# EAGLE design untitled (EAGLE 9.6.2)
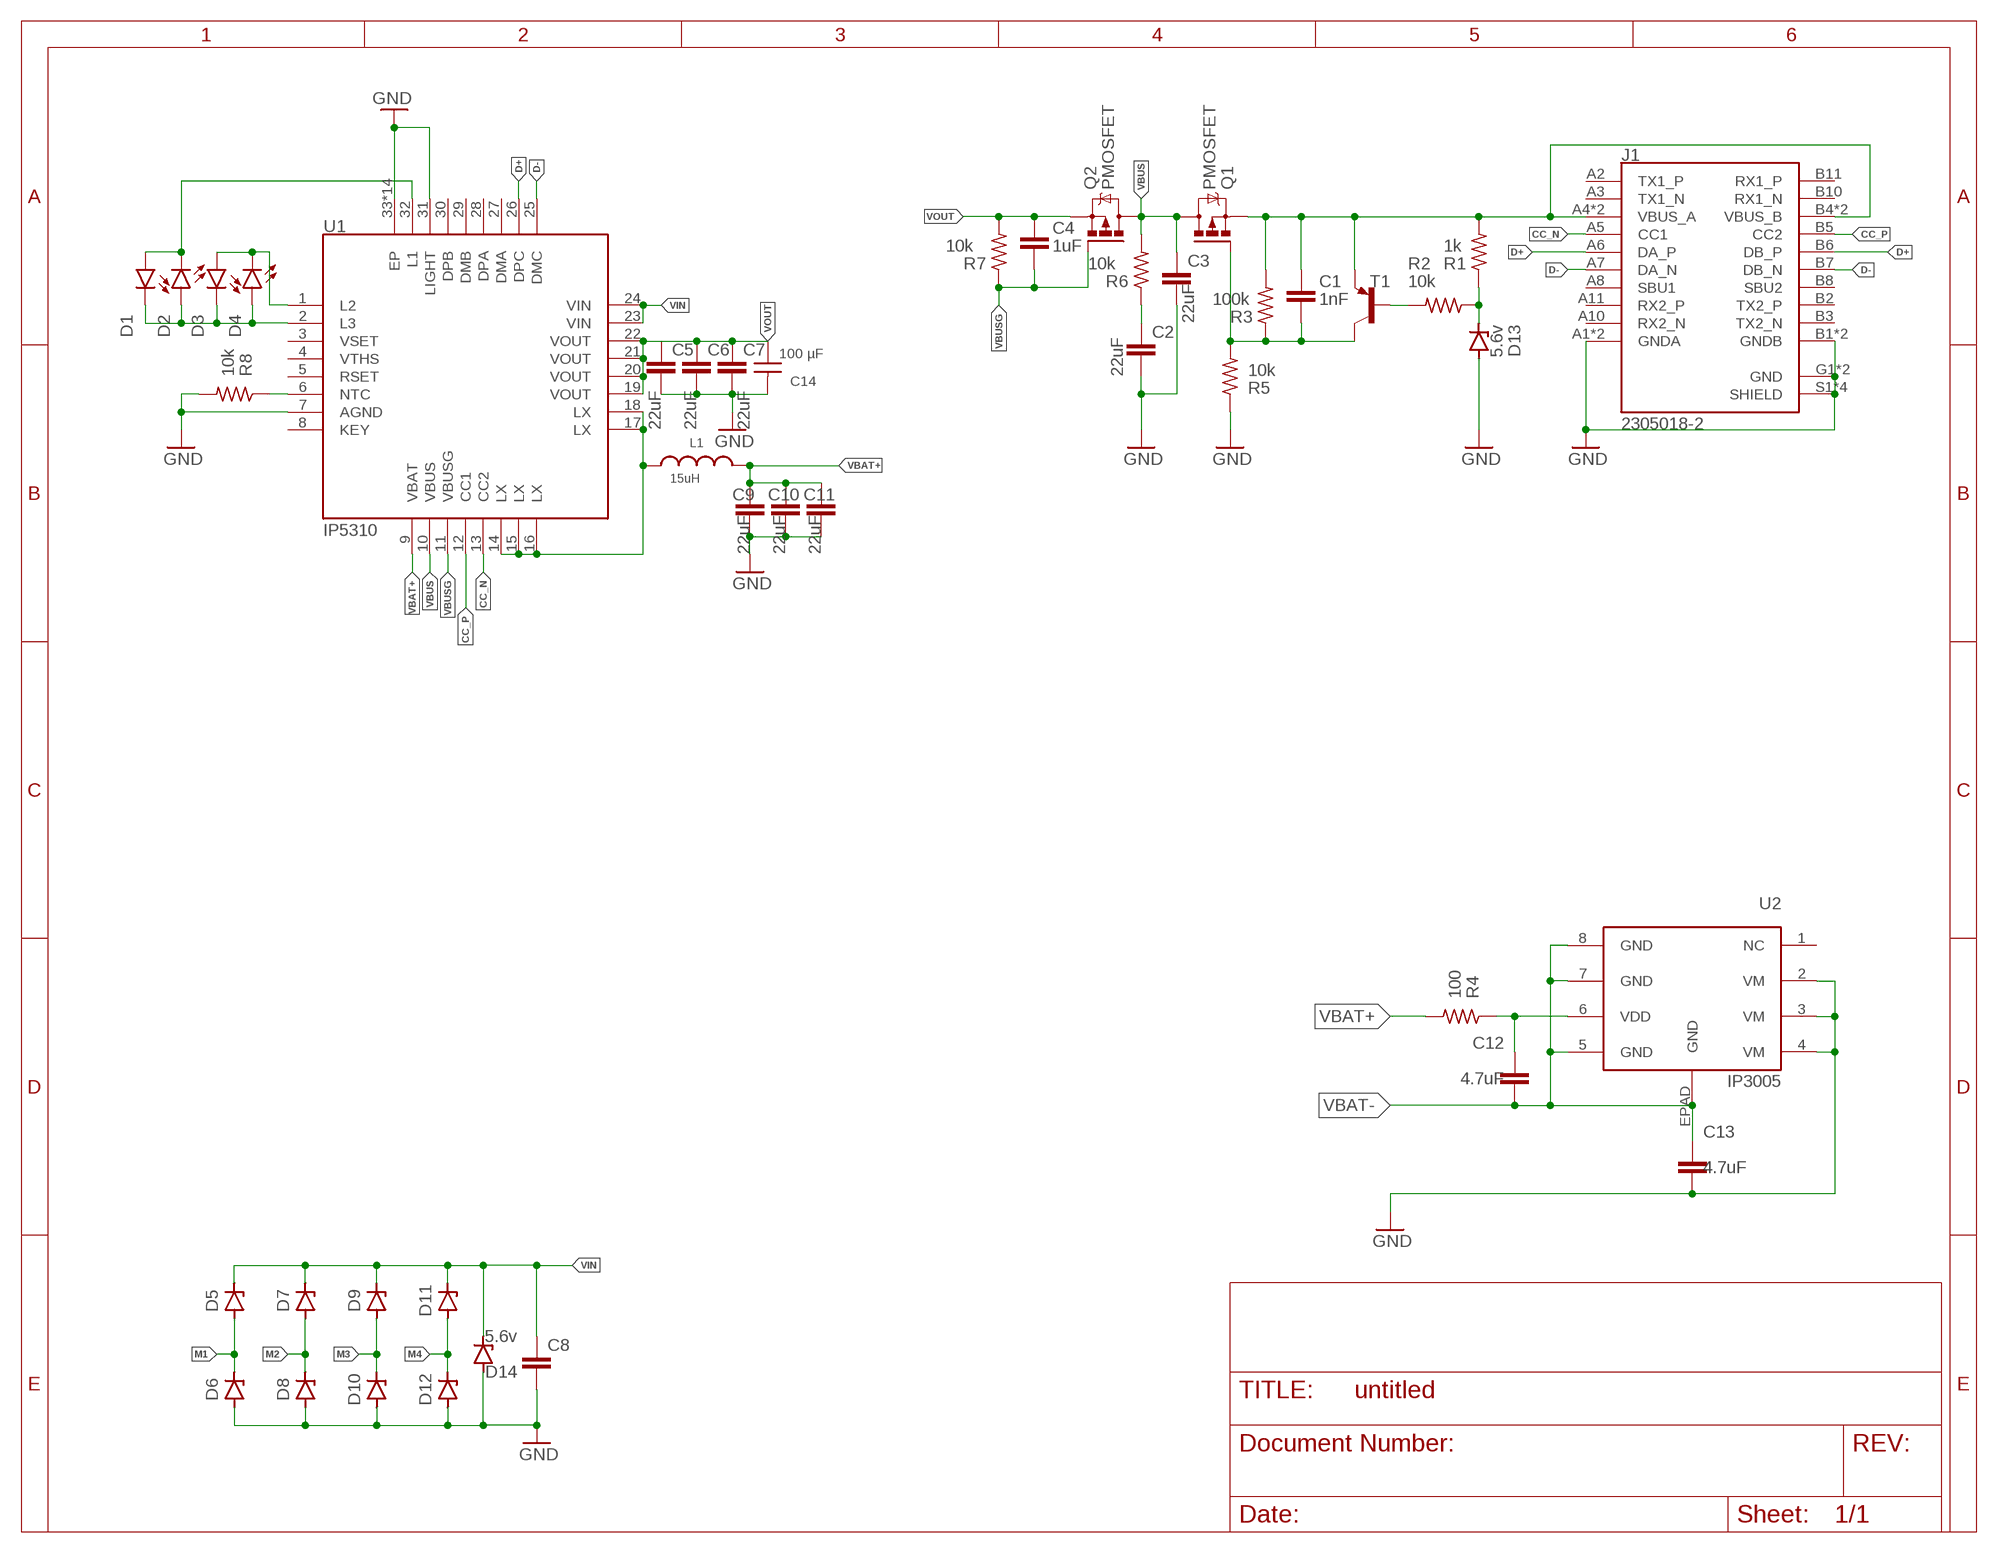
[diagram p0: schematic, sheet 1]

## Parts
C1  1nF  CC0603JRNPO9BN220  [CAP_0603]
C2  22uF  C-EUC0805  [C0805]
C3  22uF  C-EUC0805  [C0805]
C4  1uF  CC0603JRNPO9BN220  [CAP_0603]
C5  22uF  C-EUC0805  [C0805]
C6  22uF  C-EUC0805  [C0805]
C7  22uF  C-EUC0805  [C0805]
C8  C-EUC0805  [C0805]
C9  22uF  C-EUC0805  [C0805]
C10  22uF  C-EUC0805  [C0805]
C11  22uF  C-EUC0805  [C0805]
C12  4.7uF  C0603C120J5GACTU  [CAP_0603]
C13  4.7uF  C0603C120J5GACTU  [CAP_0603]
C14  100 µF  WCAP-ASNP_6.3X5.5_865250143004  [WCAP-ASNP_6.3X5.5(DXL)]
D1  LEDCHIPLED_0603  [CHIPLED_0603]
D2  LEDCHIPLED_0603  [CHIPLED_0603]
D3  LEDCHIPLED_0603  [CHIPLED_0603]
D4  LEDCHIPLED_0603  [CHIPLED_0603]
D5  ZENER_MMSZ5240BTDO-219-AB(SOD123F)  [SODFL3718X115]
D6  ZENER_MMSZ5240BTDO-219-AB(SOD123F)  [SODFL3718X115]
D7  ZENER_MMSZ5240BTDO-219-AB(SOD123F)  [SODFL3718X115]
D8  ZENER_MMSZ5240BTDO-219-AB(SOD123F)  [SODFL3718X115]
D9  ZENER_MMSZ5240BTDO-219-AB(SOD123F)  [SODFL3718X115]
D10  ZENER_MMSZ5240BTDO-219-AB(SOD123F)  [SODFL3718X115]
D11  ZENER_MMSZ5240BTDO-219-AB(SOD123F)  [SODFL3718X115]
D12  ZENER_MMSZ5240BTDO-219-AB(SOD123F)  [SODFL3718X115]
D13  5.6v  ZENER_MMSZ5240BTDO-219-AB(SOD123F)  [SODFL3718X115]
D14  5.6v  ZENER_MMSZ5240BTDO-219-AB(SOD123F)  [SODFL3718X115]
J1  2305018-2  [TE_2305018-2]
L1  15uH  WE-LHMI_7050_74437349150  [WE-LHMI_7050]
Q1  PMOSFET  PMOSFET_SOT23  [SOT23]
Q2  PMOSFET  PMOSFET_SOT23  [SOT23]
R1  1k  RC0603JR-070RL  [RES_0603]
R2  10k  RC0603JR-070RL  [RES_0603]
R3  100k  RC0603JR-070RL  [RES_0603]
R4  100  RC0603JR-070RL  [RES_0603]
R5  10k  RC0603JR-070RL  [RES_0603]
R6  10k  RC0603JR-070RL  [RES_0603]
R7  10k  RC0603JR-070RL  [RES_0603]
R8  10k  RC0603JR-070RL  [RES_0603]
T1  BC808-16-PNP-SOT23-BEC  [SOT23-BEC]
U1  IP5310  [VQFN_32]
U2  IP3005  [HSOP8]

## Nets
CC_N [cc lines]: J1.A5(CC1) U1.13(CC2)
CC_P [cc lines]: J1.B5(CC2) U1.12(CC1)
D+: J1.A6(DA_P) J1.B6(DB_P) U1.26(DPC)
D-: J1.A7(DA_N) J1.B7(DB_N) U1.25(DMC)
GND: C2.2 C3.2 C5.2 C6.2 C7.2 C8.2 C9.2 C10.2 C11.2 C13.2 C14.2 D6.2(A) D8.2(A) D10.2(A) D12.2(A) D13.2(A) D14.2(A) J1.A1(GNDA) J1.A12(GNDA) J1.B1(GNDB) J1.B12(GNDB) J1.G1(GND) J1.G2(GND) J1.S1(SHIELD) J1.S2(SHIELD) J1.S3(SHIELD) J1.S4(SHIELD) R5.1 R8.2 U1.7(AGND) U1.31(LIGHT) U1.33(EP) U1.P$1(EP) U1.P$2(EP) U1.P$3(EP) U1.P$4(EP) U1.P$5(EP) U1.P$6(EP) U1.P$7(EP) U1.P$8(EP) U1.P$9(EP) U1.P$10(EP) U1.P$11(EP) U1.P$12(EP) U1.P$13(EP) U2.2(VM) U2.3(VM) U2.4(VM)
M1: D5.2(A) D6.1(C)
M2: D7.2(A) D8.1(C)
M3: D9.2(A) D10.1(C)
M4: D11.2(A) D12.1(C)
N$1: C1.1 J1.A4(VBUS_A) J1.A9(VBUS_A) J1.B4(VBUS_B) J1.B9(VBUS_B) Q1.2(S) R1.2 R3.2 T1.E
N$2: R8.1 U1.6(NTC)
N$3: L1.1 U1.14(LX) U1.15(LX) U1.16(LX) U1.17(LX) U1.18(LX)
N$6: C2.1 R6.1
N$8: C1.2 Q1.1(G) R3.1 R5.2 T1.C
N$9: R2.2 T1.B
N$10: D1.A D2.C U1.32(L1)
N$11: D3.A D4.C U1.1(L2)
N$12: C12.1 R4.1 U2.6(VDD)
N$13: D1.C D2.A D3.C D4.A U1.2(L3)
N$14: D13.1(C) R1.1 R2.1
VBAT+: C9.1 C10.1 C11.1 L1.2 R4.2 U1.9(VBAT)
VBAT-: C12.2 C13.1 U2.5(GND) U2.7(GND) U2.8(GND) U2.EPAD(GND)
VBUS: C3.1 Q1.3(D) Q2.3(D) R6.2 U1.10(VBUS)
VBUSG: C4.2 Q2.1(G) R7.1 U1.11(VBUSG)
VIN: C8.1 D5.1(C) D7.1(C) D9.1(C) D11.1(C) D14.1(C) U1.23(VIN) U1.24(VIN)
VOUT: C4.1 C5.1 C6.1 C7.1 C14.1 Q2.2(S) R7.2 U1.19(VOUT) U1.20(VOUT) U1.21(VOUT) U1.22(VOUT)
Unconnected: J1.A2(TX1_P) J1.A3(TX1_N) J1.A8(SBU1) J1.A10(RX2_N) J1.A11(RX2_P) J1.B2(TX2_P) J1.B3(TX2_N) J1.B8(SBU2) J1.B10(RX1_N) J1.B11(RX1_P) U1.3(VSET) U1.4(VTHS) U1.5(RSET) U1.8(KEY) U1.27(DMA) U1.28(DPA) U1.29(DMB) U1.30(DPB) U2.1(NC)

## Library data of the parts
C1 C4 = Resistor_Capacitor:CC0603JRNPO9BN220: CAP CER 22PF 50V C0G/NPO 0603; CREATED_BY: PCBLayout.com; DIGIKEY_PART_NUMBER: 311-1062-2-ND; MANUFACTURER: Yageo; MPN: CC0603JRNPO9BN220; PACKAGE: SMD 0603
C2 C3 C5-C11 = resistor:C-EU: CAPACITOR, European symbol
C12 C13 = Resistor_Capacitor:C0603C120J5GACTU: CAP CER 12PF 50V C0G/NP0 0603; CREATED_BY: PCBLayout.com; DIGIKEY_PART_NUMBER: 399-1050-2-ND; MANUFACTURER: KEMET; MPN: C0603C120J5GACTU; PACKAGE: SMD 0603
C14 = Wurth_Capacitors_WCAP-ASNP:WCAP-ASNP_6.3X5.5: WCAP-ASNP Aluminium Electrolytic Capacitors; DATASHEET-URL: https://www.we-online.com/catalog/datasheet/865250143004.pdf; DF: 24%; DIAMETER: 6.3mm; I-LEAK: 14.805uA; I-RIPPLE: 45mA; L: 5.5mm; OPERATING-TEMPERATURE: -40 °C up to +85 °C; PART-NUMBER: 865250143004; TECHNICAL-REFERENCE: ASBD055470M6R3DVCTBB000; VALUE: 47 µF; VR: 6.3V(DC); Z: 0.990213Ohm
D1-D4 = led:LED: LED
D5-D14 = Diode:ZENER_: Zener Diode - Popular parts; CATEGORY: Diode; DESCRIPTION: DIODE ZENER 10V 500MW SOD123; MANUFACTURER: ON Semiconductor; MPN: MMSZ5240BT1G; SUB-CATEGORY: Zener; THERMALLOSS: 0.5W; VALUE: MMSZ5240BT1G
J1 = type-c:2305018-2: TYPE C Right Angle Sealable SMT IPX8 3.1 GEN 2 Wire to Board USB; COMMENT: 2305018-2; DESCRIPTION: USB TYPE C, REC IPX8 ON BOARD DUAL SMT; DIGI-KEY_PART_NUMBER: A132569CT-ND; MF: TE Connectivity; MP: 2305018-2; PACKAGE: None; PURCHASE-URL: https://pricing.snapeda.com/search/part/2305018-2/?ref=eda
L1 = Wurth_Power Magnetics_WE-LHMI:WE-LHMI_7050: WE-LHMI SMD Power Inductor; DATASHEET-URL: https://www.we-online.com/catalog/datasheet/74437349150.pdf; FRES: 10MHz; IR: 2.75A; ISAT: 5.5A; MOUNT: SMT; PART-NUMBER: 74437349150; RDC-MAX: 92mOhm; RDC-TYPE: 81mOhm
Q1 Q2 = Transistor:PMOSFET: P-Channel MOSFET - Generic; CATEGORY: Transistor; SUB-CATEGORY: MOSFET; TYPE: P-Channel
R1-R8 = Resistor_Capacitor:RC0603JR-070RL: RES SMD 0 OHM JUMPER 1/10W 0603; CREATED_BY: PCBLayout.com; DIGIKEY_PART_NUMBER: 311-0.0GRTR-ND; MANUFACTURER: Yageo; MPN: RC0603JR-070RL; PACKAGE: SMD 0603
T1 = transistor-neu-to92:*-PNP-: PNP Transistror
U1 = INJOINIC:IP5310
U2 = INJOINIC:IP3005

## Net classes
1 cc lines: width 0.203 mm, clearance 0.152 mm

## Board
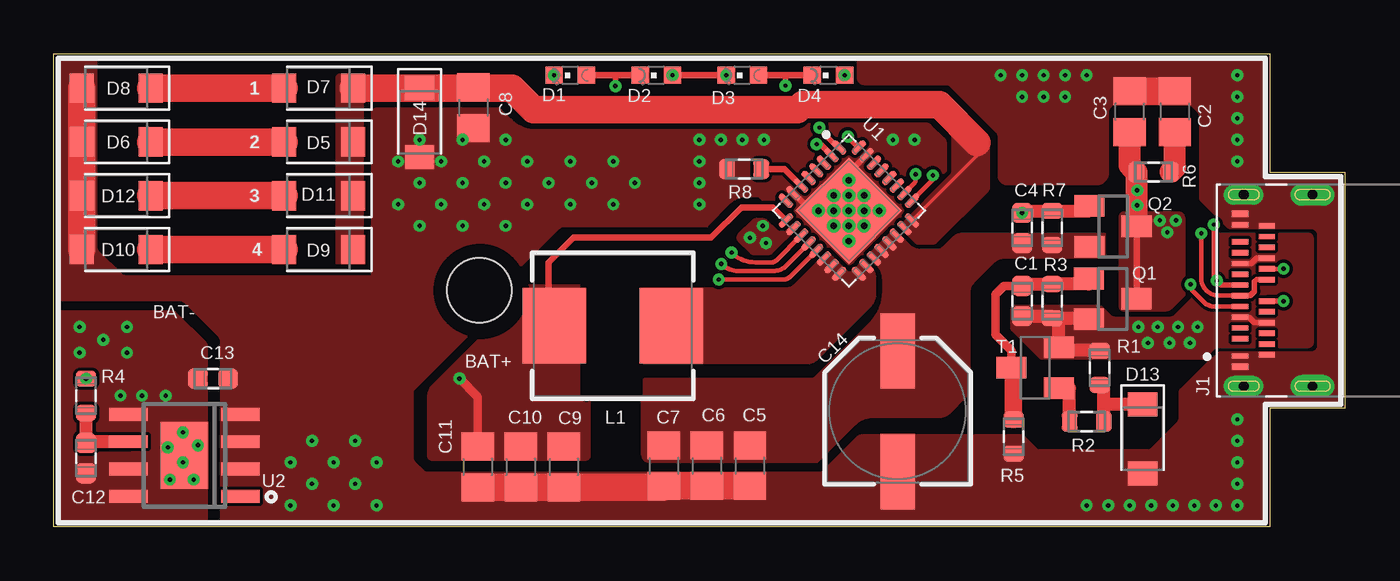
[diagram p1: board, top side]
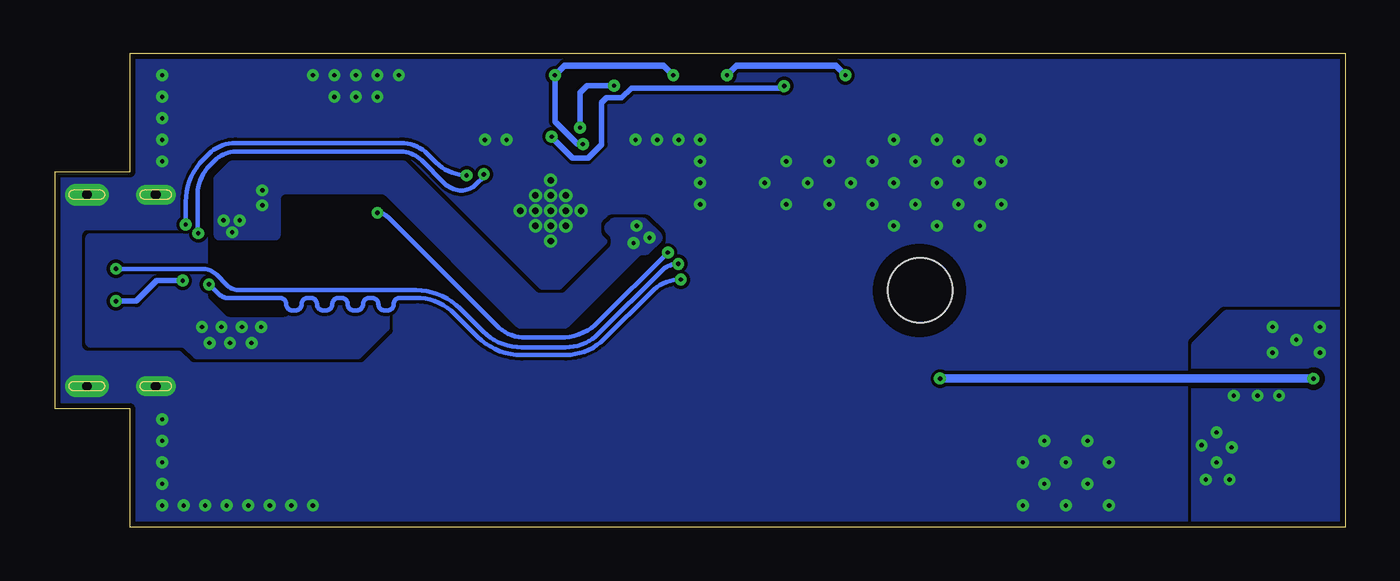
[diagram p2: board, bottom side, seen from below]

Size 60 x 22 mm. Coordinates in mm from the lower left corner, seen from the top.
Outline: 0,0 0,22 56.5,22 56.5,16.5 60,16.5 60,5.5 56.5,5.5 56.5,0 0,0
Copper layers (1*16): Top 0.035mm / dielectric 1.5mm / Bottom 0.035mm
Design rules "default *": minimum track width 6mil, minimum drill 0.1mm, track to track 6mil, track to pad 6mil, pad to pad 6mil, via to via 6mil, smd to smd 0mil, copper to edge 10mil, drill to drill 3mil, minimum pad ring 3mil, minimum via ring 3mil, stop-mask expansion 0mil, vias tented up to drill 1mm, thermal gap 10mil
Holes 3 mm at 19.78,11
tRestrict: area 53.5,11.4 to 53.6,13.3; area 52.8,11.7 to 53.1,13.6; area 18.3,9.5 to 21.3,12.5
bRestrict: area 18.3,9.5 to 21.3,12.5

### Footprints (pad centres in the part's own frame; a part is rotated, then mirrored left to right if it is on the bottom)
CAP_0603 = smd 0.92 x 0.93: 1 -0.705,0; 2 0.705,0
C0805 = smd 1.3 x 1.5: 1 -0.95,0; 2 0.95,0
WCAP-ASNP_6.3X5.5(DXL) = smd 3.5 x 1.6: 1 2.8,0; 2 -2.8,0
CHIPLED_0603 = smd 0.8 x 0.8: A 0,-0.75; C 0,0.75
SODFL3718X115 = smd 1.115 x 1.361: 1 -1.6,0; 2 1.6,0
TE_2305018-2 = smd 0.25 x 0.75: A1 -3.05,3.375; A2 -2.25,3.375; A3 -1.75,3.375; A4 -1.25,3.375; A5 -0.75,3.375; A6 -0.25,3.375; A7 0.25,3.375; A8 0.75,3.375; A9 1.25,3.375; A10 1.75,3.375; A11 2.25,3.375; A12 3.05,3.375; B1 3,2.125; B2 2.5,2.125; B3 2,2.125; B4 1.5,2.125; B5 1,2.125; B6 0.5,2.125; B7 -0.5,2.125; B8 -1,2.125; B9 -1.5,2.125; B10 -2,2.125; B11 -2.5,2.125; B12 -3,2.125 | smd 0.3 x 0.75: G1 -3.55,3.375; G2 3.55,3.375 | drill 0.45 pad 1.025 long: S1 -4.45,0; S2 4.45,0 | drill 0.45 pad 0.925 long: S3 -4.45,3.2; S4 4.45,3.2
WE-LHMI_7050 = smd 2.95 x 3.5: 1 -2.725,0; 2 2.725,0
SOT23 = smd 1 x 1.4: 1 -0.95,-1.1; 2 0.95,-1.1; 3 0,1.1
RES_0603 = smd 0.74 x 0.93: 1 -0.795,0; 2 0.795,0
SOT23-BEC = smd 1 x 1.4: B -0.95,-1.1; C 0,1.1; E 0.95,-1.1
VQFN_32 = smd 0.8 x 0.3: 1 -2.4,1.75; 2 -2.4,1.25; 3 -2.4,0.75; 4 -2.4,0.25; 5 -2.4,-0.25; 6 -2.4,-0.75; 7 -2.4,-1.25; 8 -2.4,-1.75; 17 2.4,-1.75; 18 2.4,-1.25; 19 2.4,-0.75; 20 2.4,-0.25; 21 2.4,0.25; 22 2.4,0.75; 23 2.4,1.25; 24 2.4,1.75 | smd 0.3 x 0.8: 9 -1.75,-2.4; 10 -1.25,-2.4; 11 -0.75,-2.4; 12 -0.25,-2.4; 13 0.25,-2.4; 14 0.75,-2.4; 15 1.25,-2.4; 16 1.75,-2.4; 25 1.75,2.4; 26 1.25,2.4; 27 0.75,2.4; 28 0.25,2.4; 29 -0.25,2.4; 30 -0.75,2.4; 31 -1.25,2.4; 32 -1.75,2.4 | smd 3.5 x 3.5: 33 0,0 | drill 0.3 pad 0.61: P$1 -1,1; P$2 0,1; P$3 1,1; P$4 -0.5,0.5; P$5 0.5,0.5; P$6 -1,0; P$7 0,0; P$8 1,0; P$9 -0.5,-0.5; P$10 0.5,-0.5; P$11 -1,-1; P$12 0,-1; P$13 1,-1
HSOP8 = smd 1.8 x 0.6: 1 -2.6,1.905; 2 -2.6,0.635; 3 -2.6,-0.635; 4 -2.6,-1.905; 5 2.6,-1.905; 6 2.6,-0.635; 7 2.6,0.635; 8 2.6,1.905 | smd 2.21 x 3.1: EPAD 0,0

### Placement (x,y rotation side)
C1  45,10.5 90 top
C2  52.1,19.3 90 top
C3  50,19.3 90 top
C4  45,13.9 90 top
C5  32.35,2.85 270 top
C6  30.35,2.85 270 top
C7  28.35,2.85 270 top
C8  19.5,19.5 270 top
C9  23.7,2.8 270 top
C10  21.7,2.8 270 top
C11  19.7,2.8 270 top
C12  1.5,3.2 270 top
C13  7.4,6.9 0 top
C14  39.21,5.38 90 top
D1  24,21 90 top
D2  28,21 90 top
D3  32,21 90 top
D4  36,21 90 top
D5  12.3,17.9 180 top
D6  2.9,17.9 180 top
D7  12.3,20.4 180 top
D8  2.9,20.4 180 top
D9  12.3,12.9 180 top
D10  2.9,12.9 180 top
D11  12.3,15.4 180 top
D12  2.9,15.4 180 top
D13  50.6,4.1 270 top
D14  17,18.8 270 top
J1  58.5,11 90 top
L1  25.98,9.36 180 top
Q1  49.2,10.6 270 top
Q2  49.22,13.97 270 top
R1  48.6,7.4 90 top
R2  48,4.9 180 top
R3  46.4,10.5 270 top
R4  1.5,6.1 90 top
R5  44.6,4.2 90 top
R6  51.1,16.5 180 top
R7  46.4,13.9 270 top
R8  32.08,16.64 180 top
T1  45.6,7.4 90 top
U1  36.95,14.71 315 top
U2  6.07,3.33 180 top

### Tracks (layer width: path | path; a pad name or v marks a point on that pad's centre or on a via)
CC_N  (via drill 0.2 pad 0.55)
  Top 0.203: U1.13 34.24,11.64 arc-45 33.9,11.5 v30.9,11.5 | J1.A5 53.93,10.25 arc-45 53.45,10.45 52.97,10.93 arc-45 v52.83,11.28
  Bottom 0.203: v30.9,11.5 arc-45 32.27,10.93 34.47,8.73 arc45 36.25,7.99 38.3,7.99 arc45 40.34,8.84 41.41,9.91 arc-45 43.2,10.65 43.95,10.65 arc-90 44.24,10.36 arc90 44.53,10.07 44.66,10.07 arc90 44.95,10.36 arc-90 45.25,10.65 45.38,10.65 arc-90 45.67,10.36 arc90 45.96,10.07 46.09,10.07 arc90 46.38,10.36 arc-90 46.67,10.65 46.8,10.65 arc-90 47.09,10.36 arc90 47.39,10.07 47.52,10.07 arc90 47.81,10.36 arc-90 48.1,10.65 48.23,10.65 arc-90 48.52,10.36 arc90 48.81,10.07 48.94,10.07 arc90 49.23,10.36 arc-90 49.53,10.65 51.93,10.65 arc-45 51.94,10.64 arc45 52.37,10.82 v52.83,11.28
CC_P  (via drill 0.2 pad 0.55)
  Top 0.203: v57.15,12 J1.B5 | U1.12 34.03,12.14 arc-45 33.45,11.9 31.81,11.9 arc-45 v31.01,12.23
  Bottom 0.203: v31.01,12.23 arc-45 31.8,11.9 34.72,8.98 arc45 36.25,8.35 38.3,8.35 arc45 40.09,9.09 41.16,10.16 arc-45 43.2,11.01 51.41,11.01 arc45 52,11.25 52.48,11.73 arc-45 53.14,12 v57.15,12
D+  (via drill 0.2 pad 0.55)
  Top 0.203: J1.A6 54.15,10.75 arc-90 53.32,11.58 v53.32,13.65 | v40.05,16.4 40.05,16.16 arc-45 39.97,15.95 U1.26
  Top 0.254: J1.A6 55.6,10.75 55.8,10.95 55.8,11.4 55.9,11.5 J1.B6
  Bottom 0.203: v53.32,13.65 53.35,13.68 53.35,15.47 arc45 52.8,16.8 52.55,17.05 arc45 51.6,17.45 43.9,17.45 arc45 42.95,17.05 41.87,15.97 arc-45 41.09,15.64 arc-45 40.44,15.91 40.05,16.3 v40.05,16.4
D-  (via drill 0.2 pad 0.55)
  Top 0.203: v53.91,14.06 53.9,14.05 53.9,11.81 arc45 v54.05,11.45 | v40.85,16.35 arc-45 40.7,15.98 U1.25
  Top 0.254: J1.A7 54.25,11.25 v54.05,11.45 | v57.15,10.5 J1.B7
  Bottom 0.203: v53.91,14.06 arc-45 53.9,14.07 53.9,15.11 arc45 53.09,17.09 52.83,17.34 arc45 51.6,17.85 43.9,17.85 arc45 42.67,17.34 42.27,16.94 arc-45 v40.85,16.35
  Bottom 0.254: v54.05,11.45 55.25,11.45 56.2,10.5 v57.15,10.5
GND  (via drill 0.2 pad 0.55)
  Top 0.305: U1.31 36.95,16.47 U1.P$1 | U1.7 35.18,14.71 U1.P$11
  Top 1.27: D10.2 D8.2 | C3.2 C2.2 | C11.2 C10.2 C9.2 28.3,1.85 C7.2 C6.2 C5.2
  other vias: 55,5 55,4 55,3 55,2 55,1 54,1 53,1 52,1 51,1 50,1 49,1 48,1 55,17 55,18 55,19 55,20 55,21 48,21 47,21 46,21 45,21 44,21 45,20 46,20 47,20 39,18 40,18 33,18 32,18 31,18 30,18 30,17 30,16 30,15 11,1 12,4 13,1 14,4 15,1 15,3 12,2 11,3 13,3 14,2 17,18 19,18 21,18 18,17 17,16 19,16 20,17 21,16 20,15 18,15 22,17 22,15 23,16 24,17 25,16 24,15 26,17 26,15 19,14 21,14 17,14 16,15 16,17 27,16
  pour Top (isolate 0.152, rank 2, no thermals): 7.75,-0.55 7.75,8.64 arc45 7.68,8.82 6.07,10.43 arc45 5.89,10.5 -0.85,10.5 -0.85,22.65 2,22.65 2,13.01 arc45 2.07,12.83 3.13,11.77 arc45 3.31,11.7 16.7,11.7 16.7,3.21 arc45 16.77,3.03 17.18,2.62 arc45 17.36,2.55 35.57,2.55 arc45 35.79,2.64 37.36,4.21 arc-45 37.58,4.3 44.89,4.3 arc-45 45.07,4.23 45.7,3.6 50.84,3.6 arc45 51.02,3.67 52.21,4.86 arc45 52.3,5.08 52.3,6.24 arc-45 52.37,6.42 54.03,8.08 arc-45 54.21,8.15 58.43,8.15 arc90 58.75,8.47 58.75,13.53 arc90 58.43,13.85 54.73,13.85 arc-45 54.51,13.94 53.34,15.11 arc-45 53.25,15.33 53.25,19.07 arc45 53.16,19.29 52.85,19.6 49.2,19.6 49.09,19.49 arc45 49,19.27 49,16.38 arc-45 48.91,16.16 48.74,15.99 arc-45 48.52,15.9 44.28,15.9 arc-45 44.06,15.99 43.99,16.06 arc-45 43.9,16.28 43.9,18.12 arc45 43.81,18.34 41.69,20.46 arc45 41.47,20.55 37.67,20.55 arc-90 37.35,20.87 37.35,22.65 60.4,22.65 60.4,-0.55
  pour Top (isolate 0.152, rank 2, no thermals): 16.4,6.05 20.86,10.51 arc45 20.95,10.73 20.95,11.24 arc-45 21.04,11.46 23.49,13.91 arc-45 23.71,14 30.35,14 31.46,15.11 arc-45 32.1,15.38 32.76,15.38 36.73,11.4 37.32,11.4 arc45 37.54,11.49 41.36,15.31 arc45 41.45,15.53 41.45,17.82 arc45 41.36,18.04 40.74,18.66 arc45 40.52,18.75 35.23,18.75 arc45 35.01,18.66 34.99,18.64 arc-45 34.53,18.45 22.37,18.45 arc-45 21.22,18.93 20.79,19.36 arc45 20.56,19.46 15.08,19.46 arc45 14.81,19.34 arc45 14.8,19.32 14.8,7.73 arc-45 14.71,7.51 14.34,7.14 arc-45 14.12,7.05 13.85,7.05 13.85,6 16.28,6 arc45
  pour Bottom (isolate 0.152, rank 2, no thermals): -2.4,23.6 -2.4,-3.4 arc90 -1.4,-4.4 20.6,-4.4 62.6,-4.4 arc90 63.6,-3.4 63.6,23.5 arc90 62.6,24.5 -1.5,24.5 arc90
M1
  Top 1.27: D6.1 D5.2
M2
  Top 1.27: D8.1 D7.2
M3
  Top 1.27: D10.1 D9.2
M4
  Top 1.27: D12.1 D11.2
N$1  (via drill 0.2 pad 0.55)
  Top 0.254: J1.A4 55.55,9.75 55.8,9.5 J1.B9 | J1.A9 55.65,12.25 55.9,12.5 J1.B4
  Top 0.61: R1.2 46.7,8.2 T1.E 46.7,9.71 R3.2 | C1.1 46.4,9.79 R3.2 | R3.2 48.1,9.71 Q1.2
  other vias: 50.4,9.3 51.3,9.3 52.25,9.3 50.85,8.55 51.85,8.55 53.15,9.3 52.8,8.55
  pour Top (isolate 0.152, no thermals): 44.52,9.13 45.78,7.87 arc45 45.96,7.8 53.34,7.8 arc45 53.52,7.87 53.93,8.28 arc-45 54.11,8.35 58.3,8.35 arc90 58.55,8.6 58.55,13.4 arc90 58.3,13.65 53.15,13.65 arc90 52.9,13.4 52.9,10.76 arc-45 52.83,10.58 52.07,9.82 arc-45 51.89,9.75 49.31,9.75 arc-45 49.13,9.82 48.77,10.18 arc45 48.47,10.3 44.7,10.3 arc90 44.45,10.05 44.45,9.31 arc45
  pour Bottom (isolate 0.152, no thermals): 44.52,9.13 45.78,7.87 arc45 45.96,7.8 53.34,7.8 arc45 53.52,7.87 53.93,8.28 arc-45 54.11,8.35 58.3,8.35 arc90 58.55,8.6 58.55,13.4 arc90 58.3,13.65 53.15,13.65 arc90 52.9,13.4 52.9,10.76 arc-45 52.83,10.58 52.07,9.82 arc-45 51.89,9.75 49.31,9.75 arc-45 49.13,9.82 48.77,10.18 arc45 48.47,10.3 44.7,10.3 arc90 44.45,10.05 44.45,9.31 arc45
N$2
  Top 0.305: U1.6 33.96,16.64 R8.1
N$3
  pour Top (isolate 0.152, no thermals): 27.2,7.6 35.04,7.6 arc45 35.49,7.79 38.01,10.31 arc45 38.2,10.76 38.2,11.64 arc45 38.01,12.09 37.65,12.45 37.09,11.89 arc-45 37,11.85 36.97,11.85 arc-45 36.85,11.9 35.95,12.8 34.44,11.29 arc-45 33.99,11.1 27.2,11.1
N$6
  Top 1.016: R6.1 52.1,16.7 C2.1
N$8
  Top 0.406: T1.C 44.5,8.2 43.75,8.95 43.75,10.8 44.16,11.21 C1.2
  Top 0.61: C1.2 45,11.29 R3.1 48.1,11.29 Q1.1
  Top 0.813: R5.2 44.6,7.3 T1.C
N$9
  Top 0.61: R2.2 47.2,6.45 T1.B
N$10  (via drill 0.2 pad 0.55)
  Top 0.254: U1.32 v36.9,18.15 | v26.1,20.5 26.1,21
  Top 0.305: D2.C 26.1,21 D1.A
  Bottom 0.254: v36.9,18.15 36.9,18.12 35.93,17.14 35.22,17.14 34.58,17.79 34.58,19.72 34.35,19.95 33.65,19.95 33.2,20.4 26.2,20.4 v26.1,20.5
N$11  (via drill 0.2 pad 0.55)
  Top 0.254: U1.1 36.44,17.64 35.55,18.53 v35.58,18.57 | v34,20.52 34,21
  Top 0.305: D4.C 34,21 D3.A
  Bottom 0.254: v35.58,18.57 35.58,20.19 35.25,20.52 v34,20.52
N$12
  Top 0.61: U2.6 1.56,3.96 C12.1 R4.1
N$13  (via drill 0.2 pad 0.55)
  Top 0.254: U1.2 35.63,17.8 v35.45,17.8
  Top 0.305: D3.C D2.A
  Bottom 0.254: v35.45,17.8 35.7,17.8 36.75,18.85 D4.A
  Bottom 0.305: D2.A 28.3,21.45 23.7,21.45 D1.C | D3.C 31.7,21.45 36.3,21.45 D4.A
  other vias: 23.25,21 28.75,21 31.25,21 36.75,21
N$14
  Top 0.61: R2.1 48.8,5.65 48.8,5.7 | 48.8,5.7 48.8,6.61 R1.1 | D13.1 48.8,5.7
VBAT+  (via drill 0.2 pad 0.55)
  Top 0.305: U1.9 33.41,14.85 31.95,14.85 30.55,13.45 24.15,13.45 23,12.3 23,10.9
  Top 0.406: v18.85,6.9 19.7,6.05 C11.1
  Bottom 0.406: R4.2 v18.84,6.89 v18.85,6.9
  other vias: 1.5,6.89
  pour Top (isolate 0.254, no thermals): 17.35,6.07 17.35,3.33 arc90 17.59,3.1 24.7,3.1 arc90 24.95,3.35 24.95,11 arc90 24.7,11.25 21.5,11.25 arc90 21.35,11.1 21.35,10.65 arc-45 21.14,10.14 17.55,6.55 arc45
VBAT-  (via drill 0.2 pad 0.55)
  other vias: 5.4,2.2 6.5,2.2 6,3 5.3,3.7 6.7,3.8 6,4.4 3.1,6.1 4.1,6.1 5.2,6.1 1.2,9.3 1.2,8.1 2.3,8.7 3.4,9.3 3.4,8.1
  pour Top (isolate 0.152, no thermals): -0.25,-1.9 6.9,-1.9 arc90 7.15,-1.65 7.15,2.05 7.15,8.39 arc45 7.08,8.57 5.67,9.98 arc45 5.49,10.05 -2.6,10.05 arc90 -2.85,9.8 -2.85,-0.4 -2.85,-1.65 arc90 -2.6,-1.9
  pour Bottom (isolate 0.254): -2.85,8.55 -2.85,9.8 arc-90 -2.6,10.05 5.46,10.05 arc-45 5.7,9.95 7.08,8.57 arc-45 7.15,8.4 7.15,-1.68 arc-45 7.1,-1.8 arc-45 6.86,-1.9 6.85,-1.9 -2.63,-1.9 arc-45 -2.75,-1.85 -2.78,-1.82 arc-45 -2.85,-1.65
VBUS  (via drill 0.2 pad 0.55)
  Top 0.305: Q2.3 50.32,10.65 arc-45 Q1.3
  Top 1.016: C3.1 50,16.8 R6.2 50.32,16.48 Q2.3
  other vias: 32.35,13.45 32.95,14 33.1,13.2 52.15,14.25 51.4,14.25 51.75,13.7 50.35,15.65 50.35,14.95
  pour Top (isolate 0.152, no thermals): 52.58,10.78 52.58,14.32 arc90 52.25,14.65 49.75,14.65 arc90 49.5,14.4 49.5,10.25 arc90 49.7,10.05 51.67,10.05 arc45 51.97,10.17
  pour Bottom (isolate 0.152, no thermals): 34.17,14.28 34.37,14.08 arc-90 34.37,13.72 34.22,13.57 arc45 34.15,13.39 34.15,13.16 arc45 34.22,12.98 36.28,10.92 arc45 36.46,10.85 37.44,10.85 arc45 37.62,10.92 43.63,16.93 arc-45 43.81,17 51.74,17 arc-45 51.92,16.93 52.53,16.32 arc-45 52.6,16.14 52.6,13.61 arc-90 52.35,13.36 49.75,13.36 arc-90 49.5,13.61 49.5,15.25 arc90 49.25,15.5 44.81,15.5 arc45 44.63,15.43 38.52,9.32 arc-45 38.34,9.25 36.31,9.25 arc-45 36.13,9.32 32.85,12.6 arc45 32.67,12.68 32.53,12.68 arc-45 32.35,12.75 31.83,13.27 arc-90 31.83,13.63 32.48,14.28 arc-45 32.66,14.35 33.99,14.35 arc-45
  pour Top (isolate 0.152, no thermals): 34.55,13.9 33.37,12.72 arc-45 33.19,12.65 32.56,12.65 arc-45 32.38,12.72 31.83,13.27 arc-90 31.83,13.63 32.48,14.28 arc-45 32.66,14.35 32.7,14.35 32.94,14.35 arc-45 33.12,14.28 33.55,13.85 33.58,13.82 arc45 33.76,13.75 34,13.75 34.35,14.1
VBUSG  (via drill 0.2 pad 0.55)
  Top 0.203: U1.11 33.58,12.39 arc-45 33.35,12.3 32.61,12.3 arc-45 v31.5,12.76
  Top 0.61: C4.2 45,14.7 R7.1 48.12,14.7 Q2.1
  Bottom 0.203: v31.5,12.76 34.71,9.54 arc45 36.51,8.8 38.1,8.8 arc45 39.47,9.37 44.5,14.4 arc-45 C4.2
  other vias: 45,14.61
VIN
  Top 0.152: 42.9,17.88 42.9,17.26 U1.24 | C8.1 19.45,20.4 D7.1 D14.1 | D14.1
  Top 1.27: D7.1 21.3,20.4 22.3,19.4 34.56,19.4 34.79,19.63 41.15,19.63 42.9,17.88
  pour Top (isolate 0.152, no thermals): 39.27,13.97 40.03,13.22 arc45 40.21,13.15 40.84,13.15 arc45 41.02,13.22 43.43,15.63 arc45 43.5,15.81 43.5,17.95 arc90 43.25,18.21 41.72,18.21 41.72,16.53 arc-45 41.65,16.35
  pour Top (isolate 0.254, no thermals): 13.1,12.25 14.4,12.25 14.4,21.05 13.3,21.05 arc90 13.1,20.85
VOUT
  pour Top (isolate 0.152, no thermals): 27.3,6.7 27.3,3.38 arc90 27.68,3 35.48,3 37.21,4.73 arc-45 38.11,5.1 41.19,5.1 arc45 41.64,5.29 42.41,6.06 arc45 42.6,6.51 42.6,10.94 arc-45 42.79,11.39 43.71,12.31 arc-45 44.16,12.5 48.8,12.5 arc90 48.9,12.6 48.9,13.55 arc90 48.8,13.65 42.21,13.65 arc45 41.76,13.46 41.3,13 arc-45 41.06,12.9 40.26,12.9 arc-45 39.81,13.09 39.05,13.85 37.8,12.6 38.21,12.19 arc-45 38.5,11.5 38.5,10.93 arc-45 37.92,9.52 35.34,6.94 arc-45 35.24,6.9 27.5,6.9 arc90

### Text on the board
tPlace: 1 | 2 | 3 | 4 | BAT- | BAT+

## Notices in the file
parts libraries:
Wurth_Power Magnetics_WE-LHMI: Copyright: Würth Elektronik
